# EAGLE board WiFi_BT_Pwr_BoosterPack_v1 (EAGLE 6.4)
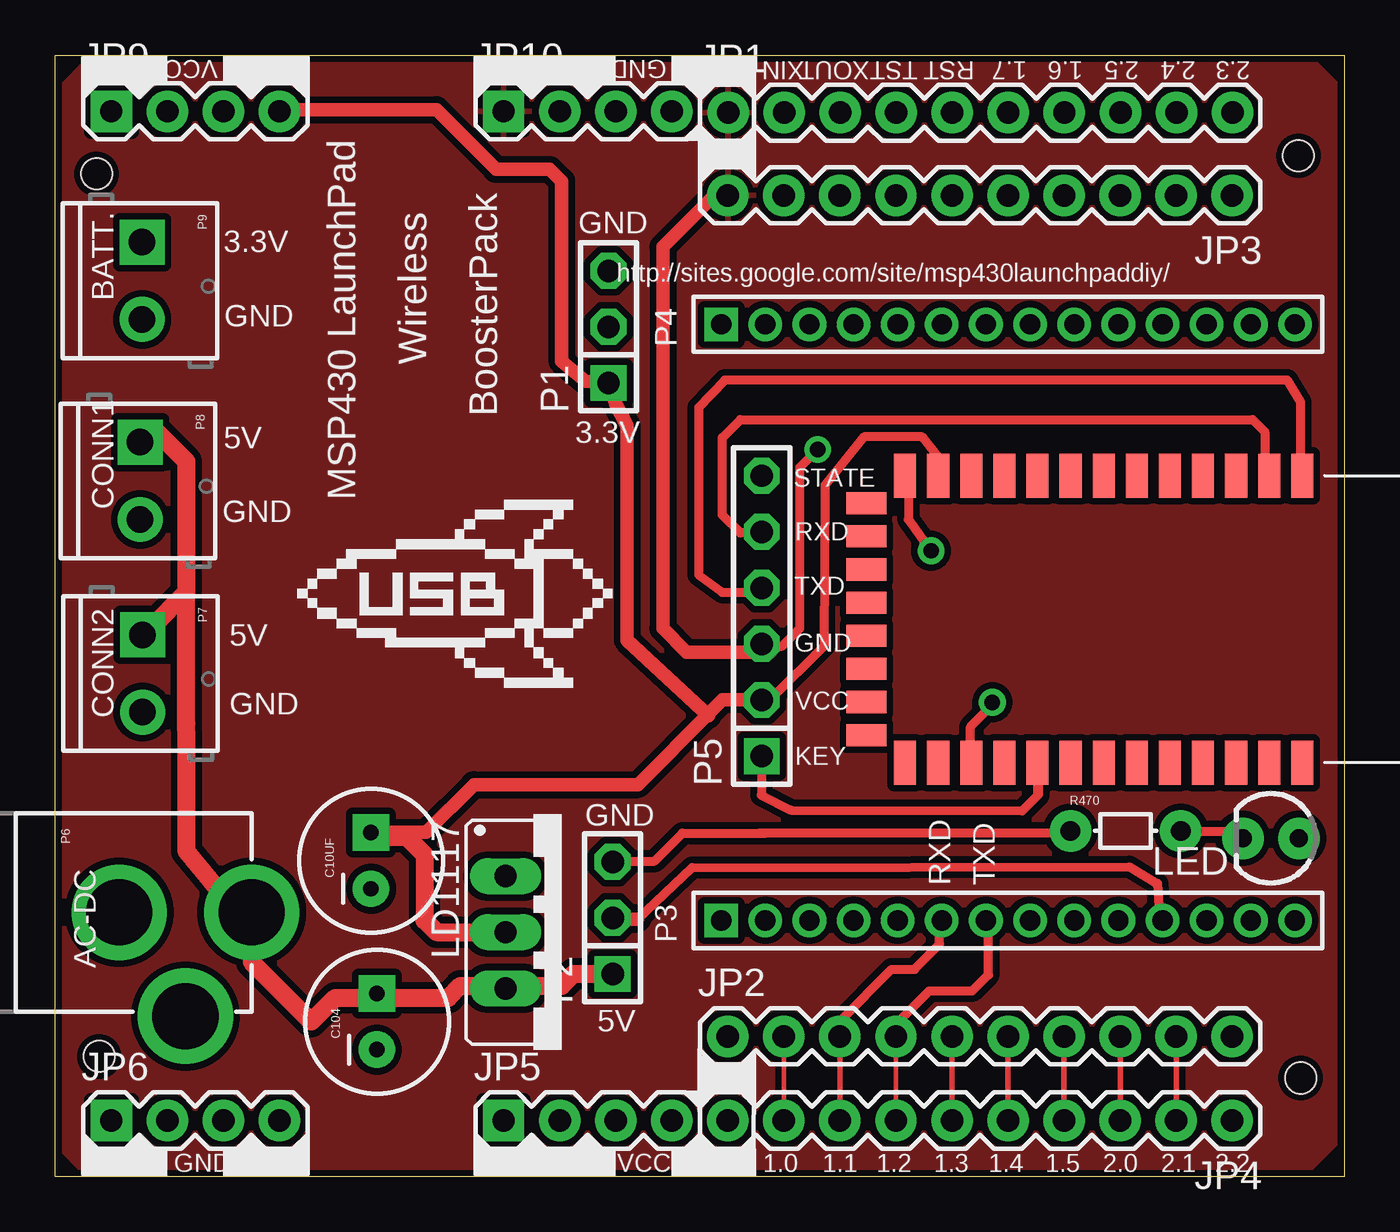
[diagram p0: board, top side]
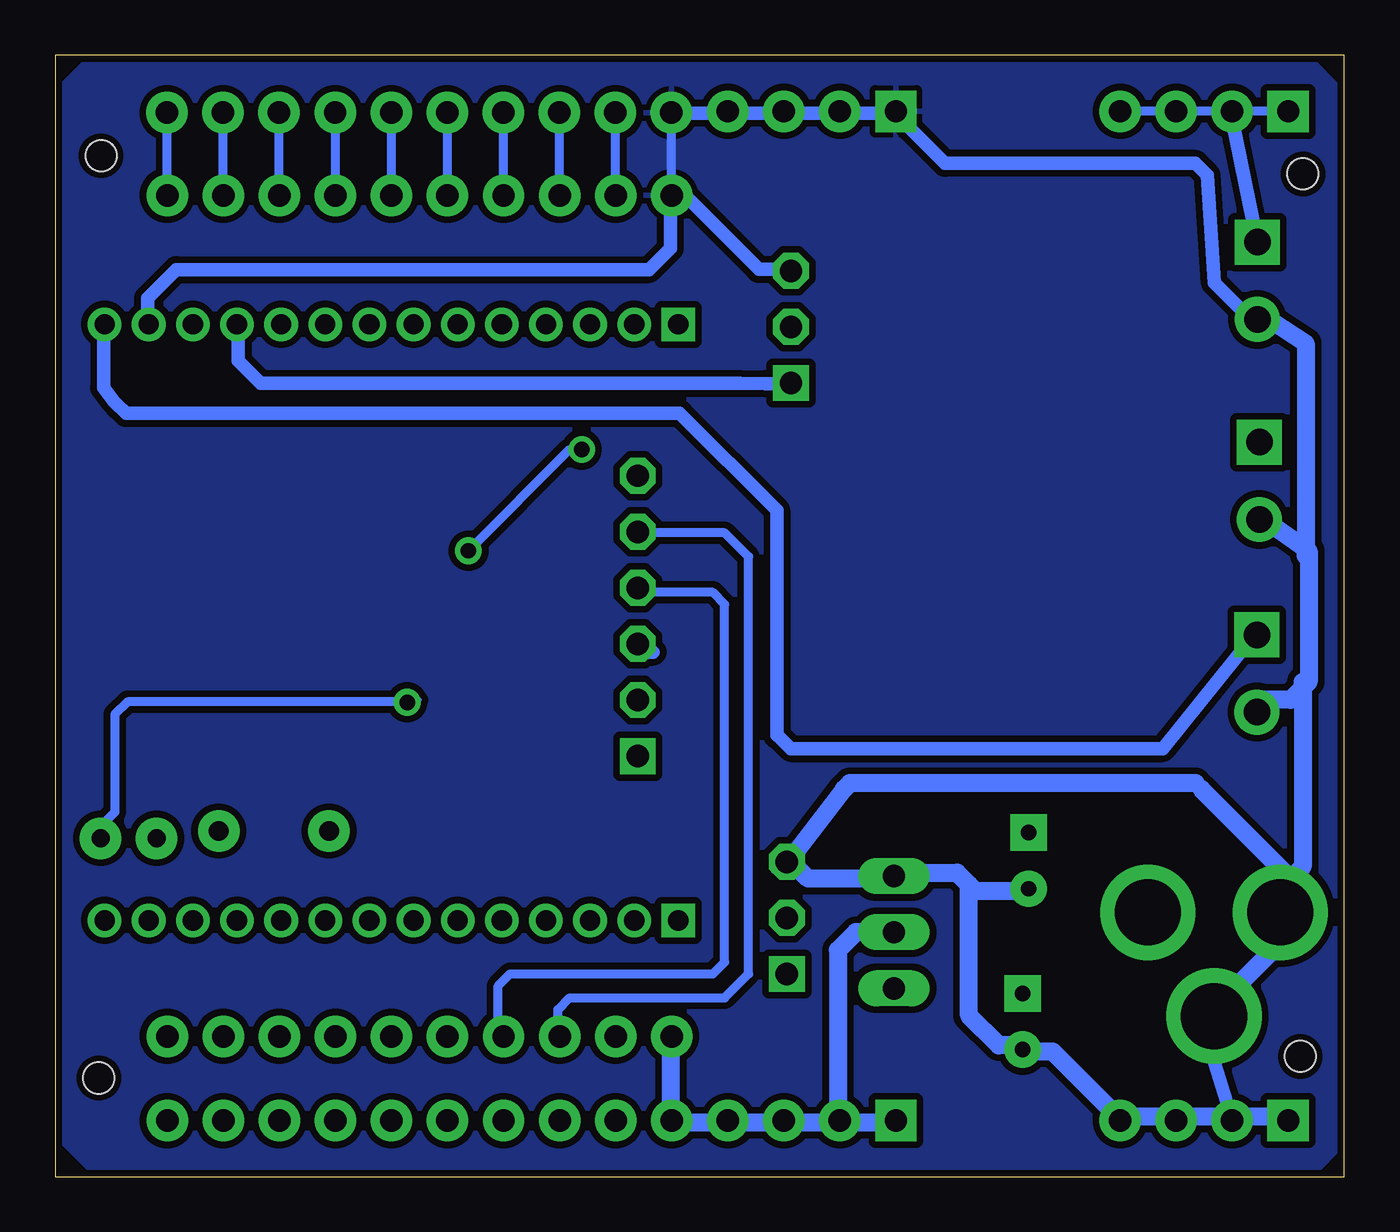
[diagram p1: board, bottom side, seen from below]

Size 58.42 x 50.8 mm. Coordinates in mm from the lower left corner, seen from the top.
Outline: 0,0 0,50.8 58.42,50.8 58.42,0 0,0
Copper layers (1*16): Top 0.035mm / dielectric 1.5mm / Bottom 0.035mm
Design rules "SparkFun": minimum track width 8mil, minimum drill 20mil, track to track 8mil, track to pad 8mil, pad to pad 8mil, via to via 8mil, smd to smd 8mil, copper to edge 10mil, drill to drill 8mil, minimum pad ring 12mil, minimum via ring 10mil, stop-mask expansion 4mil, vias tented up to drill 25mil, thermal gap 10mil
Holes 1.4 mm at 56.34,46.24 56.44,4.47 2,5.45 1.88,45.43

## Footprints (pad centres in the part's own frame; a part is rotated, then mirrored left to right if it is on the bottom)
CPOL-RADIAL-100UF-25V = drill 0.7 pad 1.651 square: 1 1.27,0 | drill 0.7 pad 1.651: 2 -1.27,0
BLUETOOTH_SMD = smd 2 x 1: 1 0,0; 2 0,-1.5; 3 0,-3; 4 0,-4.5; 5 0,-6; 6 0,-7.5; 7 0,-9; 8 0,-10.5; 9 0,-12; 10 0,-13.5; 11 0,-15; 12 0,-16.5; 13 0,-18; 22 13,-18; 23 13,-16.5; 24 13,-15; 25 13,-13.5; 26 13,-12; 27 13,-10.5; 28 13,-9; 29 13,-7.5; 30 13,-6; 31 13,-4.5; 32 13,-3; 33 13,-1.5; 34 13,0 | smd 1 x 1.8: 14 1.25,-19.75; 15 2.75,-19.75; 16 4.25,-19.75; 17 5.75,-19.75; 18 7.25,-19.75; 19 8.75,-19.75; 20 10.25,-19.75; 21 11.75,-19.75
1X10 = drill 1.016 pad 1.88: 1 0,0; 2 2.54,0; 3 5.08,0; 4 7.62,0; 5 10.16,0; 6 12.7,0; 7 15.24,0; 8 17.78,0; 9 20.32,0; 10 22.86,0
1X04 = drill 1.016 pad 1.88 square: 1 0,0 | drill 1.016 pad 1.88: 2 2.54,0; 3 5.08,0; 4 7.62,0
TO220S = drill 1.016 long: 1 -2.54,-2.54; 2 0,-2.54; 3 2.54,-2.54
LED3MM = drill 0.813 pad 1.88: A -1.27,0; K 1.27,0
1X03 = drill 1.016 square: 1 -2.54,0 | drill 1.016 octagon: 2 0,0; 3 2.54,0
1X14M = drill 0.914 square: 1 -13,0 | drill 0.914: 2 -11,0; 3 -9,0; 4 -7,0; 5 -5,0; 6 -3,0; 7 -1,0; 8 1,0; 9 3,0; 10 5,0; 11 7,0; 12 9,0; 13 11,0; 14 13,0
1X06 = drill 1.016 square: 1 -6.35,0 | drill 1.016 octagon: 2 -3.81,0; 3 -1.27,0; 4 1.27,0; 5 3.81,0; 6 6.35,0
POWER_JACK_PTH = drill 2.997 pad 4.318: GND 0,7.7; GNDBREAK 4.7,10.7; PWR 0,13.7
SCREWTERMINAL-3.5MM-2 = drill 1.2 pad 2.032 square: 1 0,0 | drill 1.2 pad 2.032: 2 3.5,0
AXIAL-5MM = drill 0.9 pad 1.88: P$1 -2.5,0; P$2 2.5,0

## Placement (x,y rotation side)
C10UF  [CPOL-RADIAL-100UF-25V]  14.31,14.31 90 top
C104  [CPOL-RADIAL-100UF-25V]  14.58,7.02 90 top
E$6  [BLUETOOTH_SMD]  56.52,31.75 270 top
JP1  M10"  [1X10]  30.49,48.2 0 top
JP2  M10"  [1X10]  30.48,6.35 0 top
JP3  M10"  [1X10]  53.34,44.45 180 top
JP4  M10"  [1X10]  53.34,2.54 180 top
JP5  [1X04]  20.32,2.54 0 top
JP6  [1X04]  2.54,2.54 0 top
JP9  [1X04]  2.54,48.26 0 top
JP10  [1X04]  20.32,48.26 0 top
LD1117  [TO220S]  22.95,11.07 270 top
LED  [LED3MM]  55.09,15.33 180 top
P1  [1X03]  25.08,38.49 90 top
P2  [1X03]  25.26,11.72 90 top
P3  [1X14M]  43.18,11.61 0 top
P4  [1X14M]  43.18,38.6 0 top
P5  [1X06]  32.02,25.4 90 top
P6  [POWER_JACK_PTH]  -4.79,11.97 270 top
P7  [SCREWTERMINAL-3.5MM-2]  3.96,24.54 270 top
P8  [SCREWTERMINAL-3.5MM-2]  3.85,33.27 270 top
P9  [SCREWTERMINAL-3.5MM-2]  3.94,42.33 270 top
R470  [AXIAL-5MM]  48.51,15.66 0 top

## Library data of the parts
C10UF C104 = SparkFun-Capacitors
E$6 = SerialPortBluetooth
JP1-JP6 JP9 JP10 = SparkFun
LD1117 = v-reg
LED = SparkFun-LED
P1-P5 = pinhead-2
P6-P9 = SparkFun-Connectors
R470 = SparkFun-Resistors

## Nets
GND: JP1.1 JP3.10 JP10.1
RST/SBWTDIO: JP1.5
S$1: JP3.8
S$2: JP3.6
S$3: JP1.7
S$4: JP1.9
S$5: JP2.3 JP4.8
S$6: JP2.2 JP4.9
S$7: JP9.1
S$8: JP3.2
S$9: JP3.4
S$10: JP6.1 JP6.4
S$11: JP2.5 JP4.6
S$13: JP3.3
S$14: JP2.1 JP4.10 JP5.1
S$20: JP3.5
S$21: JP2.4 JP4.7
S$24: JP2.6 JP4.5
S$26: JP2.9 JP4.2
S$37: JP2.7 JP4.4
S$39: P9.1
S$56: JP2.8 JP4.3
S$58: JP3.1
TEST: JP3.7
XIN: JP3.9
XOUT: JP1.3

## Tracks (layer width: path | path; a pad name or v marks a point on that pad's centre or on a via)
GND
  Bottom 0.406: JP3.10 30.48,48.26 JP10.1
  pour Top (isolate 0.305): 1.75,50.81 56.71,50.81 58.46,49.06 58.46,1.96 56.5,0 1.55,0 0,1.55 0,49.06
  pour Bottom (isolate 0.305): 1.75,50.81 56.71,50.81 58.46,49.06 58.46,1.96 56.5,0 1.55,0 0,1.55 0,49.06
RST/SBWTDIO
  Top 0.254: JP1.5 40.64,48.18
S$1
  Bottom 0.406: JP3.8 35.56,48.26
S$2
  Top 0.254: JP3.6 40.65,44.46
  Bottom 0.406: JP3.6 40.64,48.26
S$3
  Top 0.254: JP1.7 45.72,48.18
S$4
  Top 0.254: JP1.9 50.8,48.18
S$5
  Top 0.254: JP2.3 JP4.8
S$6
  Top 0.203: JP2.2 JP4.9
S$7
  Bottom 0.406: JP9.1 10.79,48.26
S$8
  Top 0.254: JP3.2 50.81,44.46
  Bottom 0.406: JP3.2 50.8,48.26
S$9
  Top 0.254: JP3.4 45.73,44.46
  Bottom 0.406: JP3.4 45.72,48.26
S$10
  Bottom 0.406: JP6.1 JP6.4
S$11
  Top 0.254: JP2.5 JP4.6
S$12
  Top 0.61: 30.24,44.28 29.7,44.28 27.54,42.12 27.54,24.84 28.62,23.76 32.4,23.76
S$13
  Top 0.254: JP3.3 48.27,44.46
  Bottom 0.406: JP3.3 48.26,48.26
S$14
  Bottom 0.254: JP2.1 JP4.10
  Bottom 0.406: JP5.1 JP4.10
S$15
  Top 0.406: 32.4,26.46 30.24,26.46 29.16,27.27 29.16,34.83 30.35,36.08 55.83,36.08 56.43,35.1 56.43,31.86
S$16
  Bottom 0.406: 35.64,6.48 35.64,7.56 35.1,8.1 28.08,8.1 27,9.18 27,28.08 28.08,29.16 31.86,29.16
S$17
  Bottom 0.406: 38.34,6.48 38.34,8.64 37.8,9.18 28.62,9.18 28.08,9.72 28.08,25.92 28.62,26.46 32.4,26.46
S$18
  Top 0.406: 31.59,29.16 31.05,29.16 30.24,29.97 30.24,33.48 31.05,34.29 54.27,34.29 54.81,33.75 54.81,32.67 55.08,32.4
S$19
  Bottom 0.61: 29.7,44.28 30.24,44.28
S$20
  Top 0.254: JP3.5 43.19,44.46
  Bottom 0.406: JP3.5 43.18,48.26
S$21
  Top 0.203: JP2.4 JP4.7
S$22
  Top 0.813: 14.04,15.39 15.93,15.39 16.74,14.58 16.74,11.61 17.28,11.07 20.25,11.07
S$23
  Bottom 0.61: 31.86,23.76 31.32,23.76
S$24
  Top 0.254: JP2.6 JP4.5
S$25
  Top 0.813: 8.91,11.88 8.91,9.72 11.61,7.02 12.69,8.1 17.82,8.1 18.36,8.64 19.44,8.64
S$26
  Top 0.254: JP4.2 JP2.9
S$27
  Bottom 0.61: 6.21,6.21 5.67,7.29
  Bottom 0.813: 5.67,7.29 5.67,7.83 2.7,10.8 2.7,13.23 | 2.7,13.23 2.7,13.77 6.48,17.55 | 1.89,22.41 1.89,14.04 2.7,13.23
S$28
  Bottom 0.61: 50.13,38.46 50.13,36.96 49.1,35.93 27.39,35.93 26.23,35.93 24.95,35.93 25.14,35.84
S$30
  Bottom 0.813: 4.25,30.23 3.98,30.02 1.62,28.35 1.62,22.41 2.43,21.6 4.05,21.6
S$31
  Bottom 0.813: 14.85,5.94 15.66,5.94 17.01,7.29 17.01,13.23 | 20.52,13.77 17.55,13.77 17.01,13.23 | 17.01,13.23 16.74,12.96 14.31,12.96
S$32
  Bottom 0.61: 5.94,7.29 6.21,6.21 5.13,2.7
S$33
  Top 0.61: 14.7,15.59 16.81,15.59 18.98,17.76 26.41,17.76 29.71,21.06
S$34
  Bottom 0.813: 14.58,5.67 13.23,5.67 10.26,2.7 | 10.26,2.7 9.99,2.43 | 2.43,2.7 10.26,2.7
S$35
  Top 0.813: 8.91,12.15 8.1,12.15 5.95,14.75 5.95,19.88 5.94,20.52 5.94,26.46 | 4.32,33.75 4.59,33.75 5.94,32.4 5.94,26.46 | 5.94,26.46 4.32,24.84
S$36
  Bottom 0.813: 20.52,13.5 24.3,13.5 25.11,14.31
S$37
  Top 0.254: JP4.4 JP2.7
S$38
  Bottom 0.813: 25.65,14.04 25.38,14.04 22.68,17.55 22.41,17.82 6.75,17.82
S$39
  Bottom 0.61: P9.1 4.9,46.96 5.13,48.06
S$40
  Bottom 0.61: 4.14,39.09 4.26,38.87 5.88,40.49 6.21,45.36 6.75,45.9 18.09,45.9 20.52,48.33
S$41
  Top 0.61: 10.53,48.33 17.28,48.33 19.98,45.63 22.41,45.63 22.95,45.09 22.95,36.94 24.04,36.03 25.14,35.99 25.07,35.89 | 25.09,35.61 25.07,35.89 | 25.07,35.89 25.39,35.01 25.92,34.02 25.92,24.3 29.6,20.88
S$42  (via drill 0.7)
  Top 0.406: 32.4,24.03 32.94,24.03 33.75,24.84 33.75,32.13 v34.56,32.94
S$43
  Top 0.406: 39.96,32.67 39.3,33.51 36.66,33.51 34.89,31.32 34.83,24.03 32.4,21.6
S$44  (via drill 0.7)
  Top 0.406: 38.66,31.09 38.66,29.78 v39.69,28.35
  Bottom 0.203: 39.37,27.94 v39.69,28.35
  Bottom 0.406: 34.83,32.94 35.1,32.94 v39.69,28.35
S$45
  Top 0.406: 32,18.96 32,17.28 33.34,16.6 43.83,16.57 44.53,17.27 44.53,17.77
S$46
  Bottom 0.813: 20.52,11.07 22.14,11.07 22.95,10.26 22.95,2.7
S$47
  Bottom 0.813: 30.51,2.43 30.51,5.94 30.78,6.21
S$48
  Bottom 0.813: 20.25,2.43 30.24,2.43
S$49
  Bottom 0.61: 54.23,38.69 54.23,39.78 52.93,41.08 31.51,41.08 30.55,42.05 30.55,44.44
S$50
  Top 0.813: 20.25,8.64 22.95,8.64 23.49,9.18 25.38,9.18
S$51
  Top 0.406: 38.17,6.4 38.17,6.97 39.61,8.41 41.56,8.41 42.29,9.14 42.29,11.67 42.34,11.72
S$52
  Top 0.406: 35.53,6.3 35.53,7.02 37.91,9.39 38.94,9.39 40.08,10.53 40.08,11.62 40.18,11.72
S$53
  Top 0.61: 31.86,21.6 30.24,21.6 29.7,21.06
S$54
  Bottom 0.813: 4,39.29 3.89,39.15 1.76,37.74 1.76,28.14 1.63,28.01
S$55
  Bottom 0.406: 25.72,19.99 25.68,19.95 25.64,19.95 | 4.04,24.59 4.23,24.65 4.23,24.57 4.14,24.48
  Bottom 0.61: 56.23,38.73 56.23,35.74 55.76,35.13 55.68,35.04 55.21,34.57 30.12,34.59 25.72,30.18 25.72,19.99 | 25.64,19.95 25.07,19.39 8.23,19.39 4.04,24.59
S$56
  Top 0.254: JP4.3 JP2.8
S$57
  Top 0.406: 26.39,11.66 28.86,13.99 48.67,14.03 49.95,13.27 50.05,11.57
  Top 0.61: 25.43,11.66 26.39,11.66 | 50.05,11.57 50.08,11.54
S$58
  Top 0.254: JP3.1 53.35,44.46
  Bottom 0.406: JP3.1 53.34,48.26
S$59
  Bottom 0.61: 30.37,44.36 29.79,44.36 26.53,41.1 25.1,41.1 25.07,41.07
S$60
  Bottom 0.61: 20.34,48.17 30.5,48.17 30.53,48.15
S$61
  Top 0.406: 44.55,18.09 44.55,17.28
S$62
  Bottom 0.406: 42.62,21.51 55.14,21.51 55.71,20.93 55.71,16.52 56.52,15.7
S$63
  Top 0.406: 53.98,15.63 51.3,15.63 51.25,15.57
S$64
  Top 0.406: 46.03,15.55 31.87,15.55
S$65
  Top 0.406: 29.84,21.17 30.09,21.43
S$66
  Top 0.406: 25.4,14.29 27.16,14.29 28.42,15.55 32.2,15.55
S$67
  Top 0.406: 42.41,21.3 41.48,20.37 41.48,19.44
S$68  (via drill 0.7)
  Bottom 0.203: 41.91,21.59 v42.47,21.49
TEST
  Top 0.254: JP3.7 38.11,44.46
  Bottom 0.406: JP3.7 38.1,48.26
XIN
  Top 0.254: JP3.9 33.03,44.46
  Bottom 0.406: JP3.9 33.02,48.26
XOUT
  Top 0.203: JP1.3 35.56,48.26

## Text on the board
tPlace: VCC | GND | XIN | XOUT | TST | RST | 1.7 | 1.6 | 2.5 | 2.4 | 2.3 | BoosterPack | Wireless | GND | 3.3V | http://sites.google.com/site/msp430launchpaddiy/ | BATT. | GND | 5V | 3.3V | MSP430 LaunchPad | STATE | CONN1 | GND | RXD | TXD | 5V | GND | CONN2 | GND | VCC | KEY | GND | RXD | TXD | AC-DC | 5V | VCC | GND | 1.0 | 1.1 | 1.2 | 1.3 | 1.4 | 1.5 | 2.0 | 2.1 | 2.2
tTest: C:/Users/wtu/Desktop/Logo_USB_LaunchPad.bmp

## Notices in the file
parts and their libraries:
SparkFun-Connectors: Licensing: CC v3.0 Share-Alike You are welcome to use this library for commercial purposes.
